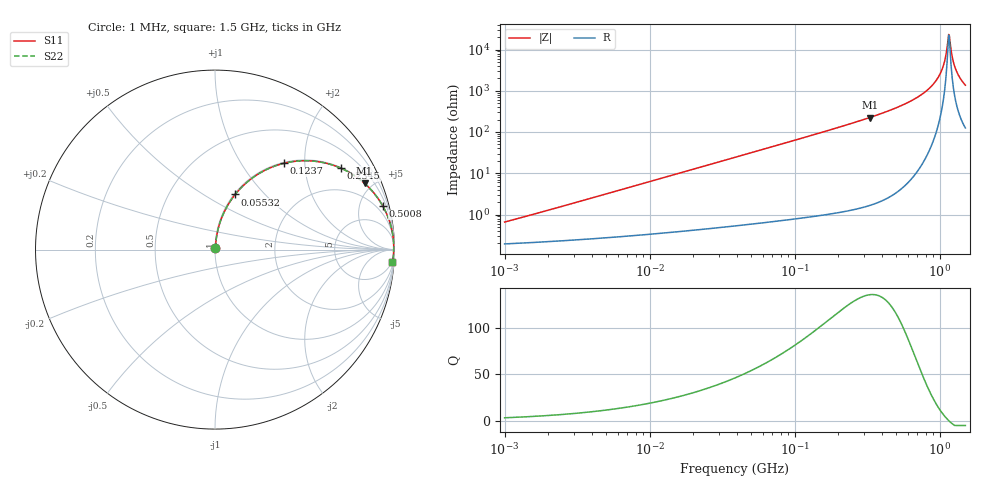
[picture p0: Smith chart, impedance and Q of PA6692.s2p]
# MHz S MA R 50
!Freq  MagS11  AngS11  MagS21  AngS21  MagS12  AngS12  MagS22  AngS22
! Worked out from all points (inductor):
!   801 points, 1 MHz to 1.5 GHz, reference 50 ohm
!   read as one part in series: L = 100 nH near 1.037 MHz
!   highest Q = 135 at 328.9 MHz (marker M1), where L = 109 nH
!   self-resonance near 1.151 GHz
!   S11 on the Smith chart (normalised r, x): 1 MHz: 1.00, +0.01; 55.32 MHz: 1.01, +0.70; 123.7 MHz: 1.02, +1.57; 234.5 MHz: 1.02, +3.07; 500.8 MHz: 1.07, +7.75; 1.5 GHz: 4, -27
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1  0.006563 72.5  0.998 -0.4  0.998 -0.4  0.006563 72.5
3.404045  0.02147 82.2  0.9973 -1.2  0.9973 -1.2  0.02147 82.2
11.48208  0.0718 83.1  0.994 -4.1  0.994 -4.1  0.0718 83.1
38.72983  0.2356 75.1  0.9668 -13.6  0.9668 -13.6  0.2356 75.1
55.31973  0.3273 69.9  0.9392 -19.1  0.9392 -19.1  0.3273 69.9
123.6659  0.6147 51.4  0.782 -37.9  0.782 -37.9  0.6147 51.4
131.8381  0.6396 49.6  0.762 -39.8  0.762 -39.8  0.6396 49.6
234.5082  0.8351 32.9  0.5434 -56.6  0.5434 -56.6  0.8351 32.9
328.8913  0.9112 23.9  0.4052 -65.7  0.4052 -65.7  0.9112 23.9
444.6989  0.9544 16.9  0.2909 -72.6  0.2909 -72.6  0.9544 16.9
500.8153  0.9663 14.4  0.2493 -75.1  0.2493 -75.1  0.9663 14.4
715.3392  0.9885 7.8  0.1356 -81.2  0.1356 -81.2  0.9885 7.8
907.2667  0.9948 3.8  0.06688 -83.7  0.06688 -83.7  0.9948 3.8
1040.607  0.996 1.6  0.0289 -81.3  0.0289 -81.3  0.996 1.6
1079.362  0.9961 1.1  0.01898 -77.5  0.01898 -77.5  0.9961 1.1
1129.842  0.9959 0.3  0.007283 -55.9  0.007283 -55.9  0.9959 0.3
1150.689  0.9958 0.1  0.004297 -14.0  0.004297 -14.0  0.9958 0.1
1182.683  0.9956 -0.4  0.007811 55.7  0.007811 55.7  0.9956 -0.4
1237.995  0.9951 -1.1  0.01959 75.0  0.01959 75.0  0.9951 -1.1
1295.894  0.9944 -1.8  0.03197 79.0  0.03197 79.0  0.9944 -1.8
1394.217  0.9929 -3.0  0.05206 80.6  0.05206 80.6  0.9929 -3.0
1500  0.9908 -4.1  0.07237 80.6  0.07237 80.6  0.9908 -4.1
